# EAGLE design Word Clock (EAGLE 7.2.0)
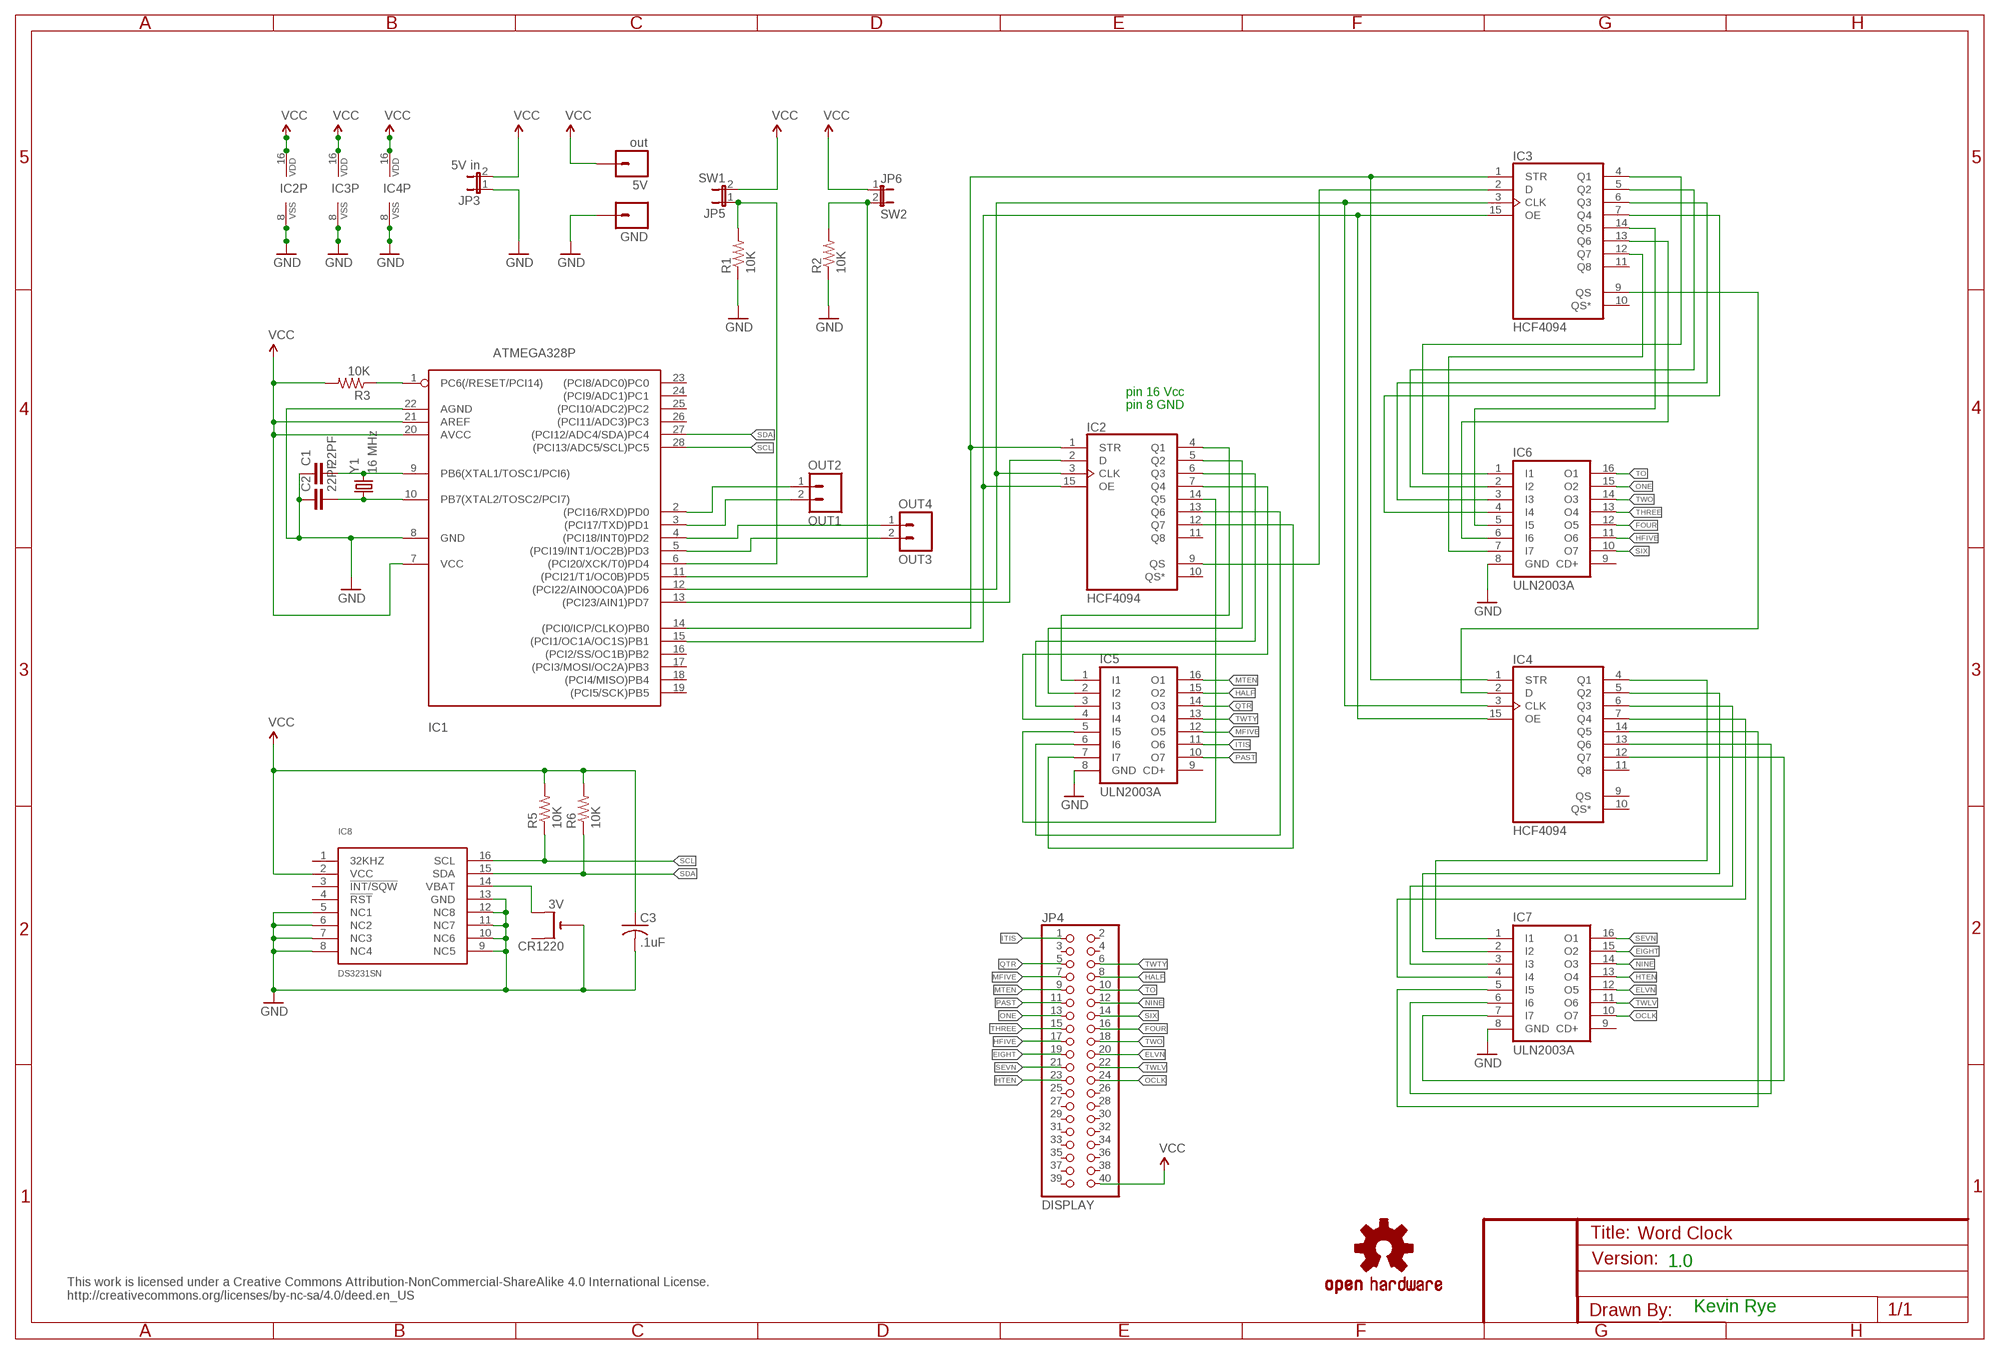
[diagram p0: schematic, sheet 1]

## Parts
5V  out  M01PTH  [1X01]
C1  22PF  CAPKIT  [CAP-PTH-SMALL-KIT]
C2  22PF  CAPKIT  [CAP-PTH-SMALL-KIT]
C3  .1uF  C-US025-024X044  [C025-024X044]
CR1220  3V  CR1220THM  [CR1220-THM]
GND  M01PTH  [1X01]
IC1  ATMEGA328P  ATMEGA168-20P  [DIL28-3]
IC2  HCF4094  4094N  [DIL16]
IC3  HCF4094  4094N  [DIL16]
IC4  HCF4094  4094N  [DIL16]
IC5  ULN2003A  ULN2003AN  [DIL16]
IC6  ULN2003A  ULN2003AN  [DIL16]
IC7  ULN2003A  ULN2003AN  [DIL16]
IC8  DS3231SN  [SO16W]
JP3  5V in  JUMPER-2PTH  [1X02]
JP4  DISPLAY  PINHD-2X20  [2X20]
JP5  SW1  JUMPER-2PTH  [1X02]
JP6  SW2  JUMPER-2PTH  [1X02]
OUT1  OUT2  M02LOCK  [1X02_LOCK]
OUT3  OUT4  M02LOCK  [1X02_LOCK]
R1  10K  RESISTORPTH-1/4W  [AXIAL-0.4]
R2  10K  RESISTORPTH-1/4W  [AXIAL-0.4]
R3  10K  RESISTORPTH-1/4W  [AXIAL-0.4]
R5  10K  RESISTORPTH-1/4W  [AXIAL-0.4]
R6  10K  RESISTORPTH-1/4W  [AXIAL-0.4]
U$2  OSHW-LOGOM  [OSHW-LOGO-M]
Y1  16 MHz  CRYSTALHC49US  [HC49US]

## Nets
EIGHT: IC7.15(O2) JP4.19
ELVN: IC7.12(O5) JP4.20
FOUR: IC6.12(O5) JP4.16
GND: C1.1 C2.1 C3.2 CR1220.- GND.1 IC1.8(GND) IC1.22(AGND) IC2.8(VSS) IC3.8(VSS) IC4.8(VSS) IC5.8(GND) IC6.8(GND) IC7.8(GND) IC8.5(NC1) IC8.6(NC2) IC8.7(NC3) IC8.8(NC4) IC8.9(NC5) IC8.10(NC6) IC8.11(NC7) IC8.12(NC8) IC8.13(GND) JP3.1 R1.P$1 R2.P$1
HALF: IC5.15(O2) JP4.8
HFIVE: IC6.11(O6) JP4.17
HTEN: IC7.13(O4) JP4.23
ITIS: IC5.11(O6) JP4.1
MFIVE: IC5.12(O5) JP4.7
MTEN: IC5.16(O1) JP4.9
N$1: IC1.14((PCI0/ICP/CLKO)PB0) IC2.1(STR) IC3.1(STR) IC4.1(STR)
N$2: IC1.13((PCI23/AIN1)PD7) IC2.2(D)
N$3: IC1.12((PCI22/AIN0OC0A)PD6) IC2.3(CLK) IC3.3(CLK) IC4.3(CLK)
N$4: IC2.4(Q1) IC5.1(I1)
N$5: IC2.5(Q2) IC5.2(I2)
N$6: IC2.6(Q3) IC5.3(I3)
N$7: IC2.7(Q4) IC5.4(I4)
N$8: IC2.14(Q5) IC5.5(I5)
N$9: IC2.13(Q6) IC5.6(I6)
N$10: IC2.12(Q7) IC5.7(I7)
N$11: IC3.4(Q1) IC6.1(I1)
N$12: IC3.5(Q2) IC6.2(I2)
N$13: IC3.6(Q3) IC6.3(I3)
N$14: IC3.7(Q4) IC6.4(I4)
N$15: IC3.14(Q5) IC6.5(I5)
N$16: IC3.13(Q6) IC6.6(I6)
N$17: IC3.12(Q7) IC6.7(I7)
N$18: IC2.9(QS) IC3.2(D)
N$19: IC1.15((PCI1/OC1A/OC1S)PB1) IC2.15(OE) IC3.15(OE) IC4.15(OE)
N$20: IC1.5((PCI19/INT1/OC2B)PD3) OUT3.2
N$22: IC4.4(Q1) IC7.1(I1)
N$23: IC4.5(Q2) IC7.2(I2)
N$24: IC4.6(Q3) IC7.3(I3)
N$25: IC4.7(Q4) IC7.4(I4)
N$26: IC4.14(Q5) IC7.5(I5)
N$27: IC4.13(Q6) IC7.6(I6)
N$28: IC4.12(Q7) IC7.7(I7)
N$29: IC3.9(QS) IC4.2(D)
N$30: CR1220.+2(+1) IC8.14(VBAT)
N$31: IC1.4((PCI18/INT0)PD2) OUT3.1
N$32: IC1.3((PCI17/TXD)PD1) OUT1.2
N$33: IC1.2((PCI16/RXD)PD0) OUT1.1
N$52: IC1.1(PC6(/RESET/PCI14)) R3.P$1
N$55: C2.2 IC1.10(PB7(XTAL2/TOSC2/PCI7)) Y1.1
N$56: C1.2 IC1.9(PB6(XTAL1/TOSC1/PCI6)) Y1.2
N$57: IC1.6((PCI20/XCK/T0)PD4) JP5.1 R1.P$2
N$58: IC1.11((PCI21/T1/OC0B)PD5) JP6.2 R2.P$2
NINE: IC7.14(O3) JP4.12
OCLK: IC7.10(O7) JP4.24
ONE: IC6.15(O2) JP4.13
PAST: IC5.10(O7) JP4.11
QTR: IC5.14(O3) JP4.5
SCL: IC1.28((PCI13/ADC5/SCL)PC5) IC8.16(SCL) R5.P$1
SDA: IC1.27((PCI12/ADC4/SDA)PC4) IC8.15(SDA) R6.P$1
SEVN: IC7.16(O1) JP4.21
SIX: IC6.10(O7) JP4.14
THREE: IC6.13(O4) JP4.15
TO: IC6.16(O1) JP4.10
TWLV: IC7.11(O6) JP4.22
TWO: IC6.14(O3) JP4.18
TWTY: IC5.13(O4) JP4.6
VCC: 5V.1 C3.1 IC1.7(VCC) IC1.20(AVCC) IC1.21(AREF) IC2.16(VDD) IC3.16(VDD) IC4.16(VDD) IC8.2(VCC) JP3.2 JP4.40 JP5.2 JP6.1 R3.P$2 R5.P$2 R6.P$2
Unconnected: CR1220.+1(+) IC1.16((PCI2/SS/OC1B)PB2) IC1.17((PCI3/MOSI/OC2A)PB3) IC1.18((PCI4/MISO)PB4) IC1.19((PCI5/SCK)PB5) IC1.23((PCI8/ADC0)PC0) IC1.24((PCI9/ADC1)PC1) IC1.25((PCI10/ADC2)PC2) IC1.26((PCI11/ADC3)PC3) IC2.10(QS*) IC2.11(Q8) IC3.10(QS*) IC3.11(Q8) IC4.9(QS) IC4.10(QS*) IC4.11(Q8) IC5.9(CD+) IC6.9(CD+) IC7.9(CD+) IC8.1(32KHZ) IC8.3(!INT/SQW) IC8.4(!RST) JP4.2 JP4.3 JP4.4 JP4.25 JP4.26 JP4.27 JP4.28 JP4.29 JP4.30 JP4.31 JP4.32 JP4.33 JP4.34 JP4.35 JP4.36 JP4.37 JP4.38 JP4.39

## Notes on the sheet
- pin 16 Vcc
- pin 8 GND
- 1.0
- This work is licensed under a Creative Commons Attribution-NonCommercial-ShareAlike 4.0 International License.
  http://creativecommons.org/licenses/by-nc-sa/4.0/deed.en_US
- Kevin Rye

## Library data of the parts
5V GND = SparkFun:M01: Header 1
C1 C2 = SparkFun:CAP: Capacitor
C3 = adafruit:C-US: CAPACITOR, American symbol
CR1220 = adafruit:CR1220: CR1216/CR1220/CR1225 12mm 3V lithium coin cell Great for battery packup. Both SMT and THM holders. Note the THM package has the ground pads on both sides of the PCB so that the masks are the same - this reduces the cost
IC1 = adafruit:ATMEGA168*P: MICROCONTROLLER 16 kBytes FLASH 1 kBytes SRAM 512 Bytes EEPROM USART 8-channel 10 bit ADC
IC2-IC4 = 40xx:4094: 8-stage SHIFT/STORE REGISTER, tri-state
IC5-IC7 = uln-udn:ULN2003A: DRIVER ARRAY
IC8 = comfile:DS3231SN
JP3 JP5 JP6 = SparkFun:JUMPER-2: Jumper
JP4 = adafruit:PINHD-2X20: PIN HEADER
OUT1 OUT3 = SparkFun:M02: Header 2
R1-R3 R5 R6 = SparkFun:RESISTOR: Resistor
U$2 = SparkFun:OSHW-LOGO: Open Source Hardware Logo This logo indicates the piece of hardware it is found on incorporates a OSHW license and/or adheres to the definition of open source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
Y1 = SparkFun:CRYSTAL: Crystals

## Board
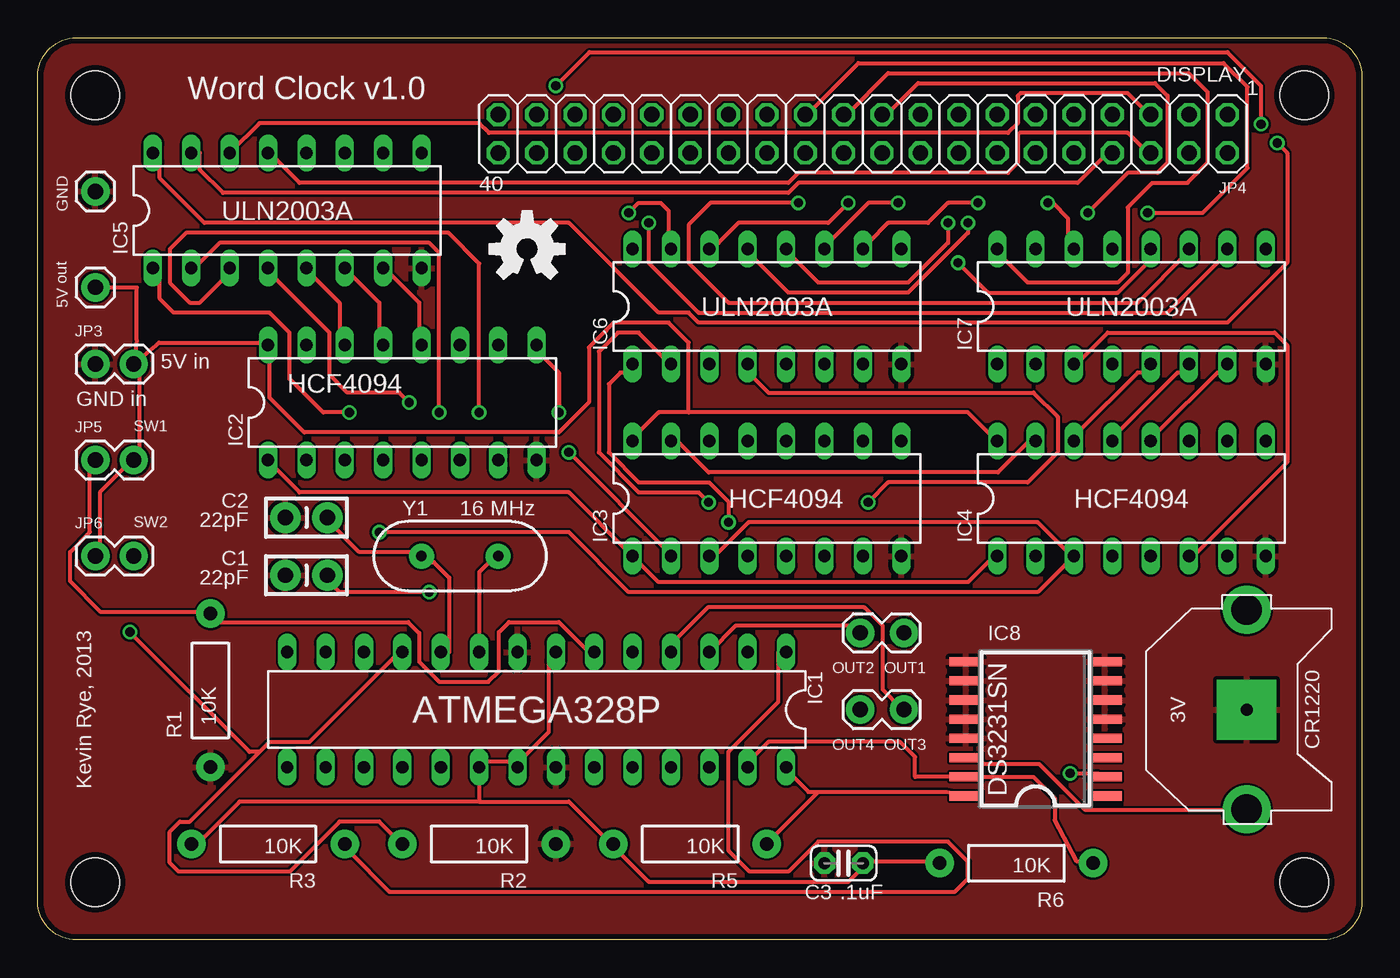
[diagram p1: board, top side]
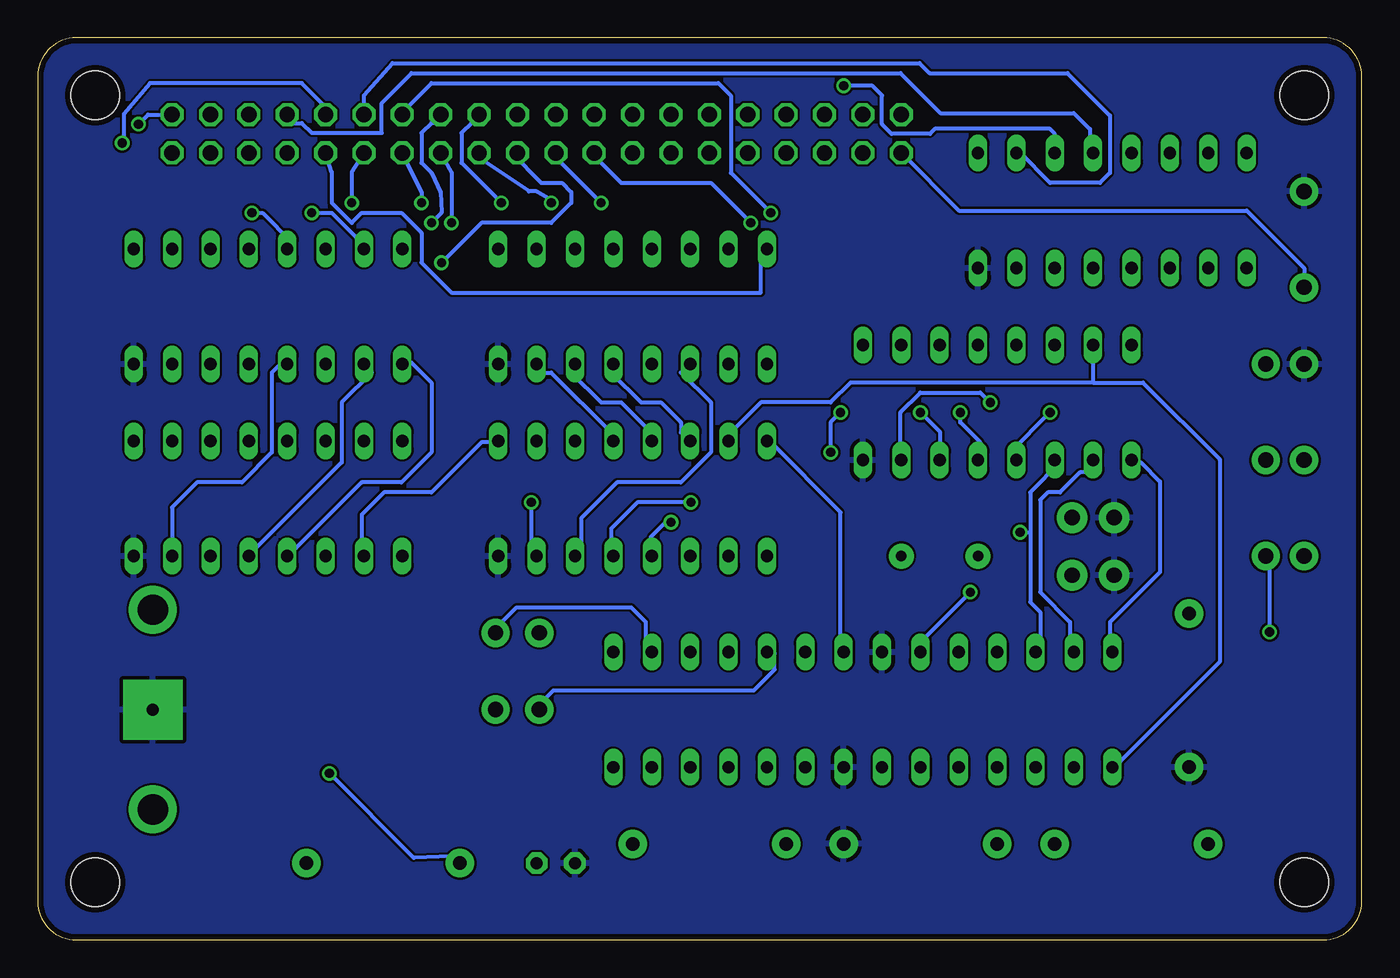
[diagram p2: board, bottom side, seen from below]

Size 87.63 x 59.69 mm. Coordinates in mm from the lower left corner, seen from the top.
Outline: 87.63,57.15 87.63,2.54 arc-90 85.09,0 2.54,0 arc-90 0,2.54 0,57.15 arc-90 2.54,59.69 85.09,59.69 arc-90 87.63,57.15
Copper layers (1*16): Top 0.0356mm / dielectric 1.5011mm / Bottom 0.0356mm
Design rules "LaenPCBOrder": minimum track width 6mil, minimum drill 13mil, track to track 6mil, track to pad 6mil, pad to pad 6mil, via to via 6mil, smd to smd 6mil, copper to edge 15mil, drill to drill 6mil, minimum pad ring 7mil, minimum via ring 7mil, stop-mask expansion 3mil, vias tented up to drill 0mil, thermal gap 10mil
Holes 3.2 mm at 3.81,55.88 3.81,3.81 83.82,3.81 83.82,55.88

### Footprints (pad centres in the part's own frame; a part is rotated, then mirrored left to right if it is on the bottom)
1X01 = drill 1.016 pad 1.88: 1 0,0
CAP-PTH-SMALL-KIT = drill 1.016 pad 2.032: 1 -1.397,0; 2 1.397,0
C025-024X044 = drill 0.813 pad 1.422 octagon: 1 -1.27,0; 2 1.27,0
CR1220-THM = drill 2 pad 3.175: +1 -6.604,0; +2 6.604,0 | drill 0.8 pad 3.962 square: - 0,0
DIL28-3 = drill 0.813 long: 1 -16.51,-3.81; 2 -13.97,-3.81; 3 -11.43,-3.81; 4 -8.89,-3.81; 5 -6.35,-3.81; 6 -3.81,-3.81; 7 -1.27,-3.81; 8 1.27,-3.81; 9 3.81,-3.81; 10 6.35,-3.81; 11 8.89,-3.81; 12 11.43,-3.81; 13 13.97,-3.81; 14 16.51,-3.81; 15 16.51,3.81; 16 13.97,3.81; 17 11.43,3.81; 18 8.89,3.81; 19 6.35,3.81; 20 3.81,3.81; 21 1.27,3.81; 22 -1.27,3.81; 23 -3.81,3.81; 24 -6.35,3.81; 25 -8.89,3.81; 26 -11.43,3.81; 27 -13.97,3.81; 28 -16.51,3.81
DIL16 = drill 0.813 long: 1 -8.89,-3.81; 2 -6.35,-3.81; 3 -3.81,-3.81; 4 -1.27,-3.81; 5 1.27,-3.81; 6 3.81,-3.81; 7 6.35,-3.81; 8 8.89,-3.81; 9 8.89,3.81; 10 6.35,3.81; 11 3.81,3.81; 12 1.27,3.81; 13 -1.27,3.81; 14 -3.81,3.81; 15 -6.35,3.81; 16 -8.89,3.81
SO16W = smd 0.6 x 2.2: 1 -4.445,-4.6; 2 -3.175,-4.6; 3 -1.905,-4.6; 4 -0.635,-4.6; 5 0.635,-4.6; 6 1.905,-4.6; 7 3.175,-4.6; 8 4.445,-4.6; 9 4.445,4.6; 10 3.175,4.6; 11 1.905,4.6; 12 0.635,4.6; 13 -0.635,4.6; 14 -1.905,4.6; 15 -3.175,4.6; 16 -4.445,4.6
1X02 = drill 1.016 pad 1.88: 1 0,0; 2 2.54,0
2X20 = drill 1.016 octagon: 1 -24.13,-1.27; 2 -24.13,1.27; 3 -21.59,-1.27; 4 -21.59,1.27; 5 -19.05,-1.27; 6 -19.05,1.27; 7 -16.51,-1.27; 8 -16.51,1.27; 9 -13.97,-1.27; 10 -13.97,1.27; 11 -11.43,-1.27; 12 -11.43,1.27; 13 -8.89,-1.27; 14 -8.89,1.27; 15 -6.35,-1.27; 16 -6.35,1.27; 17 -3.81,-1.27; 18 -3.81,1.27; 19 -1.27,-1.27; 20 -1.27,1.27; 21 1.27,-1.27; 22 1.27,1.27; 23 3.81,-1.27; 24 3.81,1.27; 25 6.35,-1.27; 26 6.35,1.27; 27 8.89,-1.27; 28 8.89,1.27; 29 11.43,-1.27; 30 11.43,1.27; 31 13.97,-1.27; 32 13.97,1.27; 33 16.51,-1.27; 34 16.51,1.27; 35 19.05,-1.27; 36 19.05,1.27; 37 21.59,-1.27; 38 21.59,1.27; 39 24.13,-1.27; 40 24.13,1.27
1X02_LOCK = drill 1.016 pad 1.88: 1 -0.178,0; 2 2.718,0
AXIAL-0.4 = drill 0.9 pad 1.88: P$1 -5.08,0; P$2 5.08,0
HC49US = drill 0.7 pad 1.651: 1 -2.54,0; 2 2.54,0

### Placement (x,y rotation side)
5V  3.81,43.18 0 top
C1  17.78,24.13 0 top
C2  17.78,27.94 0 top
C3  53.34,5.08 180 top
CR1220  80.01,15.24 270 top
GND  3.81,49.53 0 top
IC1  33.02,15.24 180 top
IC2  24.13,35.56 0 top
IC3  48.26,29.21 0 top
IC4  72.39,29.21 0 top
IC5  16.51,48.26 0 top
IC6  48.26,41.91 0 top
IC7  72.39,41.91 0 top
IC8  66.04,13.97 90 top
JP3  3.81,38.1 0 top
JP4  54.61,53.34 180 top
JP5  3.81,31.75 0 top
JP6  3.81,25.4 0 top
OUT1  57.15,20.32 180 top
OUT3  57.15,15.24 180 top
R1  11.43,16.51 90 top
R2  29.21,6.35 180 top
R3  15.24,6.35 180 top
R5  43.18,6.35 180 top
R6  64.77,5.08 180 top
U$2  32.38,45.72 0 top
Y1  27.94,25.4 0 top

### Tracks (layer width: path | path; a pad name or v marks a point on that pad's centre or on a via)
EIGHT  (via drill 0.61)
  Top 0.254: v69.49,48.11 72.14,50.75 74.12,50.75 74.78,51.41 74.78,55.87 73.95,56.69 58.27,56.69 56.29,54.71 JP4.19
  Bottom 0.254: v69.49,48.11 68.17,48.11 66.19,46.13 IC7.15
ELVN  (via drill 0.61)
  Top 0.254: v60.91,44.81 62.89,42.82 71.48,42.82 73.46,44.81 73.46,45.47 IC7.12
  Bottom 0.254: v60.91,44.81 58.27,47.45 53.64,47.45 52.32,48.77 52.32,49.48 52.94,50.09 54.3,50.09 56.29,52.07 JP4.20
FOUR  (via drill 0.61)
  Top 0.254: v60.25,47.45 60.25,46.13 57.61,43.48 51.66,43.48 49.68,45.47 IC6.12
  Bottom 0.254: v60.25,47.45 60.25,50.8 JP4.16
GND
  pour Top: 0,59.69 87.63,59.69 87.63,0 0,0
  pour Bottom: 0,0 0,59.69 87.63,59.69 87.63,0
HALF
  Top 0.254: IC5.15 10.72,52.07 10.72,50.97 12.26,49.43 49.68,49.43 50.34,50.09 68.83,50.09 70.81,52.07 JP4.8
HFIVE  (via drill 0.61)
  Top 0.254: v56.95,48.77 54.97,48.77 52.32,46.13 IC6.11
  Bottom 0.254: v56.95,48.77 59.59,51.41 59.59,53.39 58.93,54.05 JP4.17
HTEN  (via drill 0.61)
  Top 0.254: v73.46,48.11 77.11,48.11 80.06,51.06 80.06,56.44 78.48,58.01 54.3,58.01 51,54.71 JP4.23
  Bottom 0.254: v73.46,48.11 72.75,48.11 70.81,46.18 70.81,46.13 IC7.13
ITIS  (via drill 0.61)
  Top 0.254: v34.29,56.52 36.51,58.74 78.74,58.74 80.96,56.52 v80.96,53.97
  Bottom 0.254: IC5.11 20.32,53.34 20.64,53.66 28.26,53.66 28.57,53.34 31.11,53.34 31.75,53.97 31.75,55.88 32.38,56.52 v34.29,56.52 | v80.96,53.97 80.33,54.61 JP4.1
MFIVE
  Bottom 0.254: IC5.12 17.98,52.07 17.98,53.64 19.05,54.71 27.89,54.71 30.53,57.35 62.89,57.35 64.87,55.37 64.87,53.39 69.49,53.39 70.16,54.05 70.81,54.05 JP4.7
MTEN  (via drill 0.61)
  Top 0.254: v82.04,52.73 82.7,52.07 82.7,44.81 78.74,40.84 43.74,40.84 43.08,41.5 41.1,41.5 35.15,47.45 11.02,47.45 8.08,50.39 8.08,52.07 IC5.16
  Bottom 0.254: JP4.9 68.17,54.71 70.16,56.69 80.2,56.69 81.91,54.66 81.91,52.86 v82.04,52.73
N$1
  Top 0.254: IC4.1 62.89,24.99 61.57,23.67 41.1,23.67 IC3.1 35.15,29.62 17.32,29.62 15.34,31.6 IC2.1
  Bottom 0.254: IC1.14 16.66,19.05 16.66,21.03 13.36,24.33 13.36,30.33 14.63,31.6 14.68,31.6 IC2.1
N$2
  Bottom 0.254: IC1.13 19.3,19.05 19.3,21.03 21.29,23.01 21.29,29.11 20.78,29.62 19.96,29.62 18.64,30.94 17.98,30.94 17.32,31.6 IC2.2
N$3  (via drill 0.61)
  Top 0.254: IC3.3 45.06,25.65 47.04,27.63 66.19,27.63 68.17,25.65 IC4.3 66.19,23.01 39.12,23.01 35.15,26.98 v22.61,26.98
  Bottom 0.254: 21.95,26.98 21.95,29.62 19.96,31.6 IC2.3 | 21.95,26.98 21.95,22.35 21.29,21.69 21.29,19.05 IC1.12 | v22.61,26.98 21.95,26.98
N$4  (via drill 0.61)
  Top 0.254: v20.62,34.9 18.89,34.9 16.66,37.13 16.66,40.18 15.34,41.5 8.99,41.5 8.08,42.41 8.08,44.15 IC5.1
  Bottom 0.254: v20.62,34.9 23.27,32.26 IC2.4
N$5  (via drill 0.61)
  Top 0.254: v26.57,34.9 26.57,45.47 25.91,46.13 12.04,46.13 10.72,44.81 IC5.2
  Bottom 0.254: v26.57,34.9 26.57,34.24 25.25,32.92 25.25,32.26 IC2.5
N$6  (via drill 0.61)
  Top 0.254: v29.21,34.9 29.21,44.76 27.18,46.79 9.81,46.79 8.74,45.71 8.74,43.48 10.06,42.16 10.72,42.16 12.7,44.15 IC5.3
  Bottom 0.254: v29.21,34.9 27.89,33.58 27.89,32.26 IC2.6
N$7  (via drill 0.61)
  Top 0.254: v24.59,35.56 23.93,36.22 20.49,36.22 19.3,37.41 19.3,40.18 15.34,44.15 IC5.4
  Bottom 0.254: v24.59,35.56 25.25,36.22 29.21,36.22 30.53,34.9 30.53,32.26 IC2.7
N$8
  Top 0.254: IC2.14 19.96,39.52 19.96,42.16 17.98,44.15 IC5.5
N$9
  Top 0.254: IC5.6 22.61,42.16 22.61,39.52 IC2.13
N$10
  Top 0.254: IC2.12 25.25,39.52 25.25,42.16 23.27,44.15 IC5.7
N$11  (via drill 0.61)
  Top 0.254: v45.72,27.63 45.72,28.99 44.43,30.28 39.78,30.28 37.79,32.26 37.79,36.77 38.57,37.54 39.12,37.54 IC6.1
  Bottom 0.254: v45.72,27.63 46.07,27.63 47.04,26.67 47.04,25.65 IC3.4
N$12  (via drill 0.61)
  Top 0.254: v44.4,28.96 43.74,29.62 39.78,29.62 37.13,32.26 37.13,38.92 38.4,40.18 39.78,40.18 41.76,38.2 IC6.2
  Bottom 0.254: v44.4,28.96 47.93,28.96 49.68,27.21 49.68,25.65 IC3.5
N$13
  Bottom 0.254: IC3.6 51.66,25.65 51.66,27.89 49.28,30.28 45.06,30.28 43.08,32.26 43.08,35.56 45.06,37.54 IC6.3
N$14  (via drill 0.61)
  Top 0.254: v54.97,28.96 56.29,30.28 65.53,30.28 67.51,32.26 67.51,34.61 65.9,36.22 48.36,36.22 47.04,37.54 IC6.4
  Bottom 0.254: v54.97,28.96 54.97,25.65 IC3.7
N$15
  Bottom 0.254: IC3.14 45.06,33.58 45.06,34.24 46.38,35.56 47.7,35.56 49.68,37.54 IC6.5
N$16
  Bottom 0.254: IC3.13 47.04,33.58 49.02,35.56 50.34,35.56 52.32,37.54 IC6.6
N$17
  Bottom 0.254: IC3.12 49.68,33.58 53.64,37.54 54.3,37.54 IC6.7
N$18  (via drill 0.61)
  Top 0.254: v35.15,32.26 41.76,25.65 IC3.2 | v34.49,34.9 34.49,37.54 33.17,38.86 IC2.9
  Bottom 0.254: v34.49,34.9 35.15,34.24 v35.15,32.26
N$19
  Top 0.254: IC3.15 42.42,32.92 44.4,30.94 63.55,30.94 65.53,32.92 IC4.15
  Bottom 0.254: 17.78,36.88 14.48,36.88 9.4,31.8 9.4,18.39 16,11.79 IC1.15 | 17.78,36.88 17.78,38.1 17.98,38.86 IC2.15 | 17.78,36.88 33.83,36.88 35.15,35.56 39.78,35.56 41.76,33.58 IC3.15
N$20
  Bottom 0.254: IC1.5 38.86,18.95 38.86,17.88 40.23,16.51 53.49,16.51 54.71,15.29 OUT3.2
N$22
  Bottom 0.254: IC4.4 70.81,25.65 66.19,30.28 63.55,30.28 61.57,32.26 61.57,36.88 62.89,38.2 IC7.1
N$23
  Bottom 0.254: IC4.5 73.46,25.65 67.51,31.6 67.51,35.56 65.53,37.54 IC7.2
N$24
  Top 0.254: IC4.6 76.76,25.65 82.7,31.6 82.7,39.36 81.88,40.18 70.81,40.18 68.83,38.2 IC7.3
N$25
  Bottom 0.254: IC4.7 78.74,28.62 77.08,30.28 74.12,30.28 72.14,32.26 72.14,37.54 71.48,38.2 IC7.4
N$26
  Top 0.254: IC4.14 68.83,33.58 72.8,37.54 73.46,37.54 IC7.5
N$27
  Top 0.254: IC4.13 71.48,33.58 75.44,37.54 76.1,37.54 IC7.6
N$28
  Top 0.254: IC4.12 74.12,33.58 78.08,37.54 78.74,37.54 IC7.7
N$29
  Bottom 0.254: IC4.2 66.19,25.65 66.19,28.14 64.71,29.62 61.57,29.62 58.27,32.92 57.61,32.92 IC3.9
N$30
  Top 0.254: IC8.14 62.03,12.24 62.64,11.63 66.29,11.63 69.34,8.58 79.7,8.58 CR1220.+2
N$31
  Top 0.254: IC1.4 41.91,19.56 44.35,22 54.71,22 55.93,20.78 55.93,16.56 57.15,15.29 OUT3.1
N$32
  Top 0.254: IC1.3 46.18,20.78 54.1,20.78 OUT1.2
N$33
  Bottom 0.254: IC1.2 47.4,19.56 47.4,21.04 48.35,22 55.93,22 57.15,20.78 OUT1.1
N$52
  Top 0.254: IC1.1 49.02,19.05 49.02,15.75 45.72,12.45 45.72,5.91 47.11,4.52 49.68,4.52 51.66,6.5 60.25,6.5 61.57,5.18 61.57,4.06 60.71,3.2 23.27,3.2 20.62,5.84 R3.P$1
N$55
  Top 0.254: IC1.10 27.23,19.05 27.23,23.97 26.2,24.99 25.91,24.99 Y1.1 25.25,25.65 21.29,25.65 19.3,27.63 C2.2
N$56  (via drill 0.61)
  Top 0.254: IC1.9 29.21,24.33 29.87,24.99 Y1.2 | v25.91,23.01 19.96,23.01 19.3,23.67 C1.2
  Bottom 0.254: v25.91,23.01 29.21,19.71 IC1.9
N$57
  Top 0.254: IC1.6 36.47,19.05 34.49,21.03 31.19,21.03 30.53,20.37 30.53,17.78 29.82,17.07 26.57,17.07 25.25,18.39 25.25,20.3 24.52,21.03 12.04,21.03 R1.P$2 11.38,21.69 4.18,21.69 2.13,23.73 2.13,25.65 3.45,26.98 3.45,31.6 JP5.1
N$58  (via drill 0.61)
  Top 0.254: 14.68,12.45 10.06,7.82 9.4,7.82 8.74,7.16 8.74,5.1 9.32,4.52 16.66,4.52 19.96,7.82 22.61,7.82 23.93,6.5 R2.P$2 | 14.68,12.45 15.34,13.11 17.98,13.11 23.93,19.05 IC1.11 | 14.68,12.45 14.02,12.45 v6.1,20.37
  Bottom 0.254: v6.1,20.37 6.1,24.99 JP6.2
NINE  (via drill 0.61)
  Top 0.254: v66.85,48.77 67.17,48.77 68.17,47.77 68.17,46.13 IC7.14
  Bottom 0.254: v66.85,48.77 66.85,50.8 JP4.12
OCLK  (via drill 0.61)
  Top 0.254: v40.44,47.45 40.44,44.81 43.74,41.5 74.78,41.5 78.74,45.47 IC7.10
  Bottom 0.254: v40.44,47.45 43.08,50.09 49.02,50.09 51,52.07 JP4.24
ONE  (via drill 0.61)
  Top 0.254: v39.12,48.11 39.78,48.77 41.23,48.77 41.76,48.24 41.76,46.13 IC6.15
  Bottom 0.254: v39.12,48.11 41.76,50.75 41.76,55.87 42.59,56.69 61.57,56.69 63.55,54.71 JP4.13
PAST
  Bottom 0.254: IC5.10 22.61,52.07 20.62,50.09 17.32,50.09 16.66,50.75 16.66,54.55 19.47,57.35 28.6,57.35 29.26,58.01 64.16,58.01 66.04,55.88 66.04,54.71 66.19,54.71 JP4.11
QTR
  Top 0.254: IC5.14 14.68,54.05 29.21,54.05 29.87,53.39 64.21,53.39 64.87,54.05 64.87,55.85 65.05,56.03 72.14,56.03 73.46,54.71 JP4.5
SCL
  Top 0.254: 51.66,9.8 51,9.8 49.68,11.12 IC1.28 | 51.66,9.8 48.36,6.5 R5.P$1 | 51.66,9.8 60.17,9.8 IC8.16
SDA
  Top 0.254: IC1.27 47.04,11.79 48.36,13.11 57.06,13.11 58.06,12.11 58.06,10.79 IC8.15 65.89,10.79 67.31,9.37 67.31,7.92 68.78,5.18 69.49,5.18 R6.P$1
SEVN
  Top 0.254: IC7.16 63.55,45.47 65.53,43.48 71.48,43.48 72.14,44.15 72.14,48.47 73.76,50.09 76.1,50.09 77.42,51.41 77.42,56.12 76.18,57.35 56.29,57.35 53.64,54.71 JP4.21
SIX  (via drill 0.61)
  Top 0.254: v62.23,48.77 60.25,48.77 58.93,47.45 56.29,47.45 54.97,46.13 IC6.10
  Bottom 0.254: v62.23,48.77 62.23,49.48 63.55,52.07 JP4.14
THREE  (via drill 0.61)
  Top 0.254: v61.57,47.45 61.57,46.79 57.61,42.82 49.68,42.82 47.04,45.47 IC6.13
  Bottom 0.254: v61.57,47.45 60.91,48.11 60.91,48.14 60.98,49.48 61.57,50.75 62.23,51.41 62.23,53.39 61.57,54.05 60.91,54.05 JP4.15
TO
  Bottom 0.254: IC6.16 39.78,45.47 39.78,42.82 60.25,42.82 62.23,44.81 62.23,46.79 63.55,48.11 66.19,48.11 66.85,47.45 68.17,48.77 68.17,50.8 JP4.10
TWLV  (via drill 0.61)
  Top 0.254: v50.34,48.77 44.54,48.77 43.08,47.3 43.08,44.81 45.72,42.16 72.8,42.16 76.1,45.47 IC7.11
  Bottom 0.254: v50.34,48.77 53.64,52.07 JP4.22
TWO  (via drill 0.61)
  Top 0.254: v53.64,48.77 52.32,47.45 46.38,47.45 45.06,46.13 IC6.14
  Bottom 0.254: v53.64,48.77 53.34,48.77 54.61,49.53 55.12,49.53 58.93,52.07 JP4.18
TWTY
  Top 0.254: IC5.13 15.34,52.07 17.32,50.09 49.68,50.09 50.34,50.75 64.21,50.75 64.87,51.41 64.87,53.28 64.98,53.39 72.14,53.39 73.46,52.07 JP4.6
VCC  (via drill 0.61)
  Top 0.254: JP3.2 8.03,39.52 14.68,39.52 IC2.16 15.34,38.86 15.34,35.88 17.64,33.58 34.49,33.58 36.47,35.56 36.47,39.2 37.6,40.33 | JP6.1 4.12,25.65 4.12,29.62 6.1,31.6 JP5.2 6.76,32.26 6.76,37.59 JP3.2 | 43.08,34.9 61.57,34.9 62.89,33.58 IC4.16 | 43.08,34.9 41.1,34.9 39.78,33.58 IC3.16 | R6.P$2 59.59,5.18 54.97,5.18 C3.1 54.3,4.52 53.64,3.86 40.44,3.86 38.46,5.84 R5.P$2 37.79,6.5 35.15,9.14 29.21,9.14 | IC1.7 33.83,18.59 33.83,13.77 31.85,11.79 IC1.21 31.19,11.79 29.21,11.79 IC1.20 29.21,9.14 | 29.21,9.14 13.36,9.14 10.72,6.5 R3.P$2 | 37.6,40.33 38.11,40.84 41.76,40.84 43.08,39.52 43.08,34.9 | v68.33,11.02 70.16,11.02 IC8.2 | JP3.2 6.55,39.68 6.55,43.18 5V.1 | 37.64,40.28 37.6,40.33
  Bottom 0.254: IC3.16 39.12,32.92 34.49,28.3 34.49,19.05 IC1.7 | v68.33,11.02 62.74,5.44 60.2,5.54 R6.P$2 | JP4.40 26.67,48.26 7.62,48.26 3.81,44.45 5V.1

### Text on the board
Unrouted: This work is licensed under a Creative Commons Attribution-NonCommercial-ShareAlike 4.0 International License. / http://creativecommons.org/licenses/by-nc-sa/4.0/deed.en_US
tNames: Word Clock v1.0 | 1 | 40 | GND in | C2 | 22pF | C1 | 22pF | Kevin Rye, 2013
